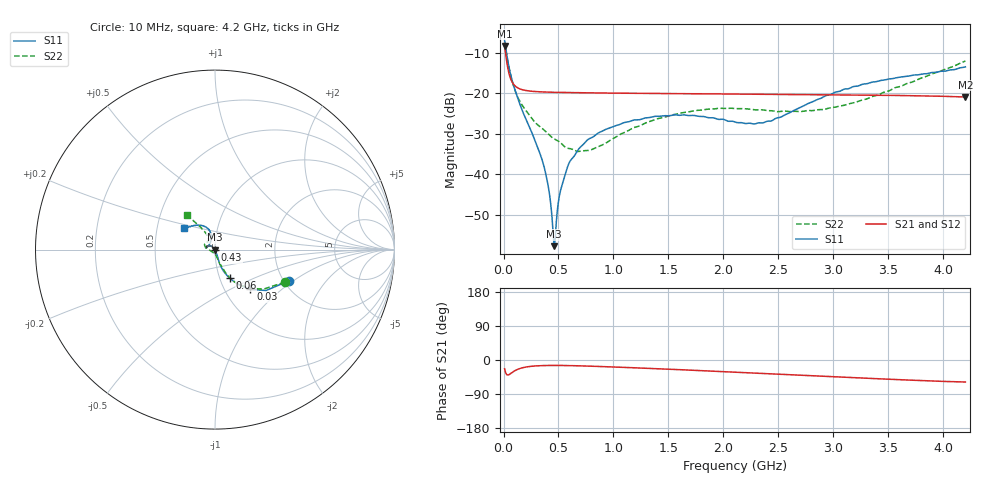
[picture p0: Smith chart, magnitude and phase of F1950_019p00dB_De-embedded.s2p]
! Integrated Device Technology
! Corporate Headquarters
! 6024 Silver Creek Valley Road
! San Jose, CA 95138  USA
! Phone:  1-408-284-8200
! Toll Free:  1-800-223-1366
! Webpage:  http://www.idt.com/
! Timing and RF Division
! 515 Groton Road, Suite 102
! Westford, MA 01886-6024
! Device:  F1950
! Description: 7-bit 0.25 dB Digital Step Attenuator
! Frequency:  150.0 -  4000.00 MHz
! Package:  4x4 mm Thin QFN Plastic Package: 24 pin
! Ports:  2 RF, 12 DC
!  Pin  1  = D0
!  Pin  2  = VDD
!  Pin  3  = Vmode
!  Pin  4  = GND
!  Pin  5  = RF1  =  Port 1
!  Pin  6  = GND
!  Pin  7  = GND
!  Pin  8  = GND
!  Pin  9  = GND
!  Pin 10  = GND
!  Pin 11  = GND
!  Pin 12  = GND
!  Pin 13  = GND
!  Pin 14  = RF2  =  Port 2
!  Pin 15  = GND
!  Pin 16  = LE
!  Pin 17  = CLK
!  Pin 18  = DATE
!  Pin 19  = D6
!  Pin 20  = D5
!  Pin 21  = D4
!  Pin 22  = D3
!  Pin 23  = D2
!  Pin 24  = D1
! State:  76
! Atten State:  19.00 dB
! Voltage:  +5.00 Volts
! Current:  Not Measured mA
! Data:  The device was measured on a the F195X evaluation board which has
!  individual transmission lines to the RF pins.  Data was collected
!  using a calibrated network analyzer.  The evaluation board was
!  de-embedded using a TRL calibration technique.
!  The reference plane is the edge of the package pin.
! Misc:  Board 2019
!  Action Tracker AT0250
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# GHz S dB R 50
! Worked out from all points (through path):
!   420 points, 10 MHz to 4.2 GHz, reference 50 ohm
!   highest |S21| = -8.40 dB at 10 MHz (marker M1); lowest = -20.9 dB at 4.2 GHz (marker M2)
!   group delay of S21, straight-line fit = 30.2 ps
!   lowest |S11| = -57.6 dB at 460 MHz (marker M3), VSWR 1.00, Z = 49.9 - j0.0838 ohm
!   |S11| at or under -10 dB: 26.88 MHz to end of sweep
!   |S22| runs from -34.3 to -7.3 dB; largest |S21 - S12| = 0.00017
!   S11 on the Smith chart (normalised r, x): 10 MHz: 2.11, -0.92; 30 MHz: 1.31, -0.64; 60 MHz: 1.12, -0.37; 430 MHz: 1.00, -0.01; 4.2 GHz: 0.69, +0.17
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0.01  -7.02 -23.2  -8.40 -23.4  -8.40 -23.4  -7.32 -24.9
0.03  -10.56 -48.4  -12.36 -38.8  -12.36 -38.8  -10.86 -48.6
0.06  -14.96 -62.6  -16.09 -36.9  -16.09 -36.9  -14.97 -62.2
0.15  -22.80 -71.8  -18.95 -22.4  -18.95 -22.4  -22.07 -71.3
0.35  -36.31 -68.8  -19.69 -14.8  -19.69 -14.8  -28.61 -80.0
0.4  -41.92 -72.0  -19.74 -14.4  -19.74 -14.4  -29.84 -81.5
0.43  -47.39 -82.0  -19.76 -14.3  -19.76 -14.3  -30.61 -83.9
0.45  -53.81 -103.0  -19.78 -14.3  -19.78 -14.3  -31.06 -86.6
0.46  -57.64 -140.2  -19.78 -14.3  -19.78 -14.3  -31.24 -88.1
0.48  -51.75 150.9  -19.79 -14.3  -19.79 -14.3  -31.52 -90.6
0.5  -46.61 140.3  -19.81 -14.3  -19.80 -14.4  -31.81 -92.3
0.52  -43.78 138.6  -19.82 -14.4  -19.81 -14.4  -32.22 -93.4
0.57  -39.18 134.0  -19.84 -14.6  -19.84 -14.6  -33.41 -101.3
0.71  -33.01 137.4  -19.89 -15.6  -19.89 -15.6  -34.22 -126.1
0.99  -28.26 147.0  -19.98 -18.3  -19.98 -18.4  -31.29 -168.9
1.41  -25.68 162.9  -20.08 -23.2  -20.08 -23.2  -26.22 168.4
1.73  -25.48 168.3  -20.14 -27.2  -20.14 -27.2  -24.33 159.6
2.11  -27.14 157.9  -20.21 -32.3  -20.21 -32.3  -23.79 150.4
2.43  -26.85 126.0  -20.27 -36.3  -20.27 -36.4  -24.31 141.0
2.81  -22.12 105.0  -20.34 -41.6  -20.34 -41.6  -24.29 126.5
3.51  -16.49 117.2  -20.53 -50.8  -20.52 -50.9  -19.37 119.6
4.2  -13.52 145.8  -20.93 -58.1  -20.93 -58.2  -12.10 129.5
